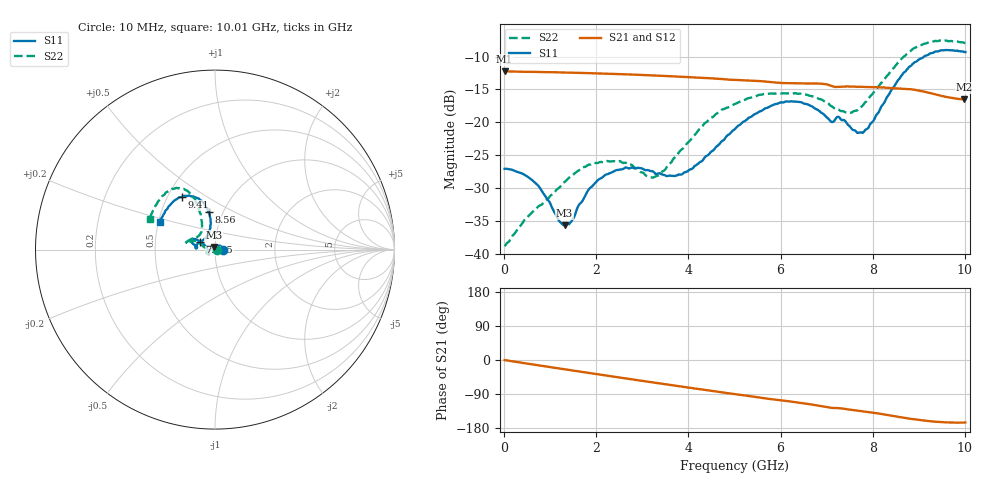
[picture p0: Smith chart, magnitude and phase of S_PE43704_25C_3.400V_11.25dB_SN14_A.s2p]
! Device ID: PE43704
! Dir: z:\PE43704\PE43704_Char_1_20130516\PE43704\AMB\3p400V\11p25dB
! Serial: 14
! Insertion: A
! Impedance: 50 ohm
! Temp: Amb
! VDD: 3.400V
! Attenuation Step: 11.25dB
! IDD: 1.140487e-01mA
#  Hz  S  RI  R  50
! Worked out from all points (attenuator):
!   401 points, 10 MHz to 10.01 GHz, reference 50 ohm
!   highest |S21| = -12.25 dB at 10 MHz (marker M1); lowest = -16.5 dB at 9.985 GHz (marker M2)
!   lowest |S11| = -35.7 dB at 1.31 GHz (marker M3), VSWR 1.03, Z = 49.2 + j1.45 ohm
!   |S11| at or under -10 dB: start of sweep to 9.115 GHz
!   |S22| runs from -38.8 to -7.5 dB; largest |S21 - S12| = 0.0017
!   S11 on the Smith chart (normalised r, x): 10 MHz: 1.09, +0.00; 7.485 GHz: 0.84, +0.07; 8.56 GHz: 0.86, +0.37; 9.41 GHz: 0.59, +0.39; 10.01 GHz: 0.51, +0.18
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1e7  0.0443 0.000231  0.2442 -0.00087  0.2443 -0.000865  0.0114 0.000359
6.85e8  0.0266 0.0217  0.2355 -0.0542  0.2356 -0.0541  -0.00285 0.0217
1.31e9  -0.00748 0.0147  0.2177 -0.0991  0.2177 -0.099  -0.0328 0.0128
1.46e9  -0.0151 0.00917  0.2121 -0.109  0.2121 -0.1089  -0.0384 0.0072
1.685e9  -0.0248 0.000637  0.2029 -0.1235  0.2029 -0.1234  -0.045 -0.00214
2.01e9  -0.0338 -0.0113  0.1876 -0.1426  0.1876 -0.1424  -0.047 -0.0137
2.41e9  -0.0367 -0.0223  0.1663 -0.1635  0.1665 -0.1633  -0.046 -0.0208
3.16e9  -0.0344 -0.0255  0.1211 -0.1931  0.1212 -0.1929  -0.0369 -0.0101
3.36e9  -0.035 -0.0213  0.108 -0.1988  0.1081 -0.1986  -0.0395 -0.00355
4.035e9  -0.0437 0.00239  0.0628 -0.2111  0.0632 -0.2109  -0.0694 0.0218
4.46e9  -0.0545 0.02  0.0345 -0.2142  0.0346 -0.2142  -0.0971 0.0435
5.01e9  -0.0784 0.0421  -0.000244 -0.2101  -0.000181 -0.2103  -0.1303 0.046
5.96e9  -0.1266 0.06  -0.054 -0.1925  -0.0532 -0.1927  -0.1593 0.0456
6.685e9  -0.1271 0.036  -0.0918 -0.175  -0.0919 -0.1747  -0.1503 0.0486
7.485e9  -0.0851 0.0409  -0.1221 -0.142  -0.122 -0.1421  -0.0883 0.0811
7.835e9  -0.0474 0.0735  -0.1344 -0.1282  -0.1344 -0.1285  -0.0733 0.1219
8.36e9  -0.0247 0.1629  -0.1514 -0.1024  -0.1508 -0.1028  -0.087 0.2195
8.56e9  -0.0352 0.2086  -0.1571 -0.0898  -0.1563 -0.0899  -0.1063 0.2665
8.935e9  -0.0818 0.2768  -0.162 -0.0687  -0.1619 -0.0675  -0.165 0.3323
9.41e9  -0.1843 0.293  -0.1549 -0.0463  -0.155 -0.0459  -0.2562 0.3264
9.985e9  -0.301 0.1625  -0.1443 -0.0383  -0.1447 -0.0384  -0.3592 0.1792
1.001e10  -0.3063 0.1528  -0.145 -0.039  -0.1455 -0.0389  -0.3629 0.1704
